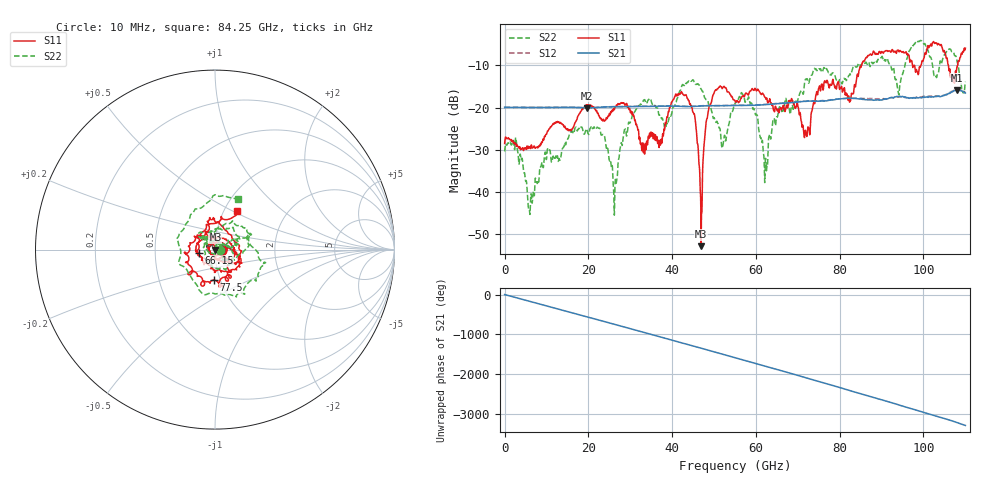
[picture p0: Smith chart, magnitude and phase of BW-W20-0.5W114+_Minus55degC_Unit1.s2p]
!Mini-Circuits Laboratory
!S-Parameters
!Model: BW-W20-0.5W114+
!Run / Lot / Date Code: QN2409253 /  / N/A
!Fixture:
!Network Analyzer: PNA-X N5242B - 423 4 ports (COM/DCOM);  Serial number: 74408
!Date: 3/8/2024 at 1:32:54 PM
!No.: Unit# 1 (U1  -55C)
!Tested with:
# Hz  S  dB  R  50
!Frequency  S11 dB  S11 Deg  S21 dB  S21 Deg  S12 dB  S12 Deg  S22 dB  S22 Deg
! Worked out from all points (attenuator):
!   2208 points, 10 MHz to 110 GHz, reference 50 ohm
!   highest |S21| = -15.90 dB at 108 GHz (marker M1); lowest = -20.1 dB at 19.75 GHz (marker M2)
!   lowest |S11| = -52.8 dB at 46.9 GHz (marker M3), VSWR 1.00, Z = 50.2 - j0.0563 ohm
!   |S11| at or under -10 dB: start of sweep to 85.21 GHz; 97.35 GHz to 99.36 GHz (2.011 GHz wide, 2.04 % of centre); 106 GHz to 108.1 GHz (2.193 GHz wide, 2.05 % of centre)
!   |S22| runs from -45.5 to -4.1 dB; largest |S21 - S12| = 0.15
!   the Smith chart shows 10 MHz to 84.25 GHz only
!   S11 on the Smith chart (normalised r, x): 10 MHz: 1.08, -0.00; 66.15 GHz: 0.83, -0.03; 77.5 GHz: 0.93, -0.33; 84.25 GHz: 1.15, +0.53
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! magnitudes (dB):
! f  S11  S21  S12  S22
! 10 MHz  -28.5  -19.9  -19.9  -30.4
! 6.1 GHz  -29.4  -20.0  -19.9  -44.8
! 18.35 GHz  -20.7  -20.0  -20.0  -24.6
! 19.75 GHz  -19.4  -20.1  -20.0  -25.6
! 26.4 GHz  -19.8  -19.8  -19.8  -37.6
! 31 GHz  -22.8  -19.8  -19.7  -21.1
! 36.7 GHz  -27.7  -19.7  -19.6  -21.0
! 43.25 GHz  -17.0  -19.7  -19.7  -14.3
! 45.3 GHz  -21.5  -19.7  -19.7  -14.1
! 46.9 GHz  -52.8  -19.6  -19.6  -15.5
! 49.95 GHz  -16.7  -19.6  -19.5  -22.4
! 52.3 GHz  -15.0  -19.6  -19.5  -27.7
! 55.05 GHz  -18.5  -19.5  -19.4  -19.0
! 58.65 GHz  -16.1  -19.5  -19.4  -19.0
! 62.3 GHz  -17.8  -19.3  -19.2  -32.0
! 66.15 GHz  -20.6  -19.0  -18.9  -20.9
! 73.35 GHz  -20.9  -18.5  -18.4  -12.3
! 77.5 GHz  -15.4  -18.3  -18.2  -11.8
! 84.25 GHz  -12.1  -17.9  -17.8  -10.2
! 91.7 GHz  -6.6  -17.8  -17.8  -9.4
! 108 GHz  -10.3  -15.9  -15.8  -9.2
! 110 GHz  -5.9  -16.6  -16.4  -13.9
